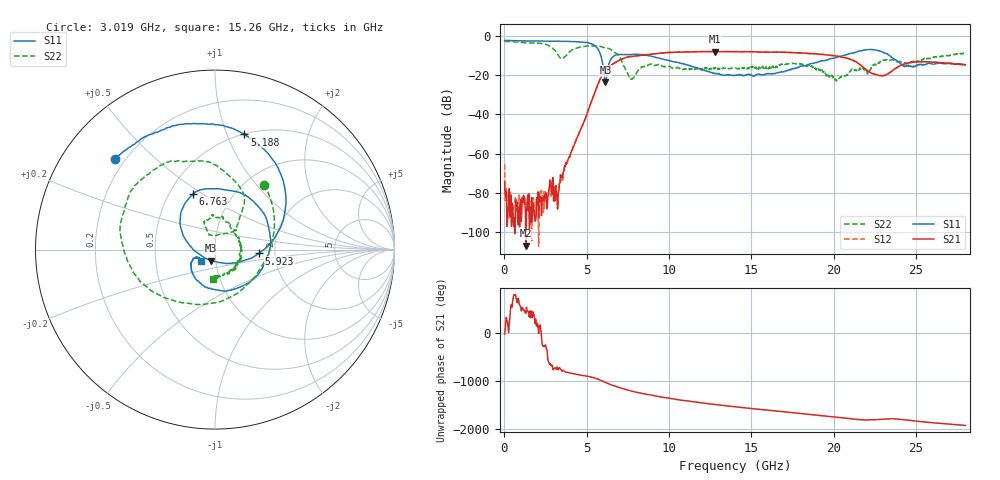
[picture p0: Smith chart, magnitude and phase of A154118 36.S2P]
!  2-Port S-parameters saved by WinCal
! VAR MeasName=S-Parameters (CALIBRATED_DATA) read from VNA (N5230A)
! VAR MeasDate=2015-9-10 14:37:11
! VAR NAME=A154118 36
! VAR FILENAME=A154118 36.S2P
! VAR DATE=2015-9-10 14:37:11
! VAR PHYS_PORTS=1,2
# Hz S DB R 50
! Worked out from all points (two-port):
!   801 points, 10 MHz to 28 GHz, reference 50 ohm
!   highest |S21| = -7.81 dB at 12.78 GHz (marker M1); lowest = -107.2 dB at 1.305 GHz (marker M2)
!   |S21| within 3 dB of the highest: 7.414 GHz to 20.62 GHz (13.21 GHz wide, 94.2 % of centre)
!   lowest |S11| = -23.6 dB at 6.133 GHz (marker M3), VSWR 1.14, Z = 47.6 - j5.99 ohm
!   |S11| at or under -10 dB: 5.857 GHz to 6.673 GHz (816.2 MHz wide, 13 % of centre); 8.77 GHz to 20.54 GHz (11.77 GHz wide, 80.3 % of centre); 23.41 GHz to end of sweep
!   |S22| runs from -22.9 to -2.7 dB; largest |S21 - S12| = 0.0083
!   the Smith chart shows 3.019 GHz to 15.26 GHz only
!   S11 on the Smith chart (normalised r, x): 3.019 GHz: 0.16, +0.38; 5.188 GHz: 0.51, +1.16; 5.923 GHz: 1.65, -0.08; 6.763 GHz: 0.65, +0.45; 15.26 GHz: 0.85, -0.11
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1e7  -2.15 179.7  -74.59 -21.1  -65.40 92.6  -2.67 179.8
1.849375e8  -2.16 177.2  -90.75 -118.8  -84.94 -4.9  -2.69 175.5
1.304538e9  -2.36 162.8  -107.17 51.9  -85.82 42.8  -3.36 148.5
2.494112e9  -2.46 146.3  -82.66 112.7  -84.85 61.2  -4.13 102.5
3.018925e9  -2.51 137.9  -79.44 -12.4  -80.58 -36.3  -6.86 53.0
3.718675e9  -2.61 124.4  -64.83 -88.3  -64.87 -79.0  -10.07 -102.8
4.698325e9  -3.01 98.1  -46.47 -159.7  -46.41 -158.6  -5.29 166.2
5.18815e9  -3.58 75.6  -35.55 172.5  -35.53 172.6  -4.88 143.1
5.922888e9  -12.19 -5.0  -20.04 86.6  -19.99 86.8  -5.41 112.5
6.132812e9  -23.64 -108.0  -17.30 53.2  -17.23 53.0  -5.92 101.5
6.762588e9  -9.58 112.0  -13.26 -28.5  -13.23 -28.8  -8.58 67.9
7.70725e9  -9.34 72.3  -10.33 -124.6  -10.30 -124.8  -21.78 94.2
9.351662e9  -11.09 -27.7  -8.82 121.2  -8.74 121.1  -14.52 78.5
1.117101e10  -14.95 -134.7  -8.02 25.1  -7.93 24.4  -16.81 19.6
1.278044e10  -18.96 -157.1  -7.81 -44.2  -7.80 -45.0  -16.15 -45.6
1.4005e10  -19.94 -149.4  -7.90 -91.6  -7.90 -92.2  -16.47 -79.4
1.526455e10  -19.98 -142.0  -7.96 -137.3  -7.95 -137.7  -15.80 -94.9
1.869332e10  -13.87 -115.4  -8.88 106.3  -8.88 105.9  -15.32 -135.1
2.019779e10  -10.69 -122.9  -10.21 53.5  -10.12 52.7  -22.10 -120.4
2.334666e10  -9.68 170.2  -18.93 18.6  -19.00 17.4  -12.43 -100.1
2.43613e10  -15.28 178.4  -13.97 -4.2  -13.98 -5.1  -13.76 -110.4
2.8e10  -14.69 -156.3  -14.59 -119.4  -14.67 -120.2  -8.41 -112.2
